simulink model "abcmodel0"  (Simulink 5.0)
settings: Solver=ode45  StartTime=0.0  StopTime=2  RelTol=1e-3
InitFcn:
  | imparamsim0
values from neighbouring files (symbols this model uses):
  Bm = 0.10    (= 0.1)    [IMabc2.m]    (also in imabcparam.m = 0.01; IMabcrun0.m = 0.01; IMabcrun1.m = 0.001; IMcur0.m = 1e-06)
  gam = 2*pi/3    (= 2.09439510239)    [IMabc2.m]    (also in IMabcf0.m; IMabcf1.m; imabcparam.m; IMabcrun0.m)
  J = 0.02    [imabcparam.m]    (also in IMabcrun0.m; IMabcrun1.m; imdefSIvec1.m = 0.03)
  Lm1 = 2/3*Lm    [IMabcf0.m]    (also in IMabcf1.m; imabcparam.m = 0.0564666666667; IMabcrun0.m = 0.0564666666667; IMabcrun1.m = 0.0564666666667)
  Lrr = [Lr   -Lm/2 -Lm/2    [IMabc2.m]    (also in IMabcf0.m = [Lr   -Lm1/2 -Lm1/2; IMabcf1.m = [Lr   -Lm1/2 -Lm1/2)
  Lss = [Ls   -Lm/2 -Lm/2    [IMabc2.m]    (also in IMabcf0.m = [Ls   -Lm1/2 -Lm1/2; IMabcf1.m = [Ls   -Lm1/2 -Lm1/2)
  nsync = 120*freq0/p    (= 1800)    [imabcparam.m]
  p = cos(beta-alpha)    [abcRwdg.m]    (also in alternator.m = 0:pi/20:2*pi; altwdgs.m = 0:pi/20:2*pi; brushlessdcB.m = 0:pi/100:2*pi; brushlessdcnew.m = 0:pi/100:2*pi)
  R = str2num(get(h,'string'))    [acttrcalc1.m]    (also in IMabc2.m = diag([Rs Rs Rs Rr Rr Rr]); IMabcf0.m = diag([Rs Rs Rs Rr Rr Rr]); IMabcf1.m = diag([Rs Rs Rs Rr Rr Rr]); IMcurf0.m = diag([Rs Rs Rr Rr]))
  Vs = abs(Vas)    [calc0.m]    (also in Ccurverun.m = 1; IMabc2.m = 1; IMabcrun0.m = Vll*sqrt(2/3); IMabcrun1.m = Vll*sqrt(2/3))
  wk = ws    (= 1)    [imdef0vec.m]    (also in imdef1vec.m; imdef2vec.m; imdefrotflux.m; imdefSIvec1.m)
  wo = 2*pi*freq0    [calc0.m]    (also in IMabc2.m = 376.991118431; imabcparam.m = 376.991118431; IMabcrun0.m = 376.991118431; IMabcrun1.m = 376.991118431)
undefined symbols (not defined in the file or in its folder): TL1, TL2
libraries: simulink x17

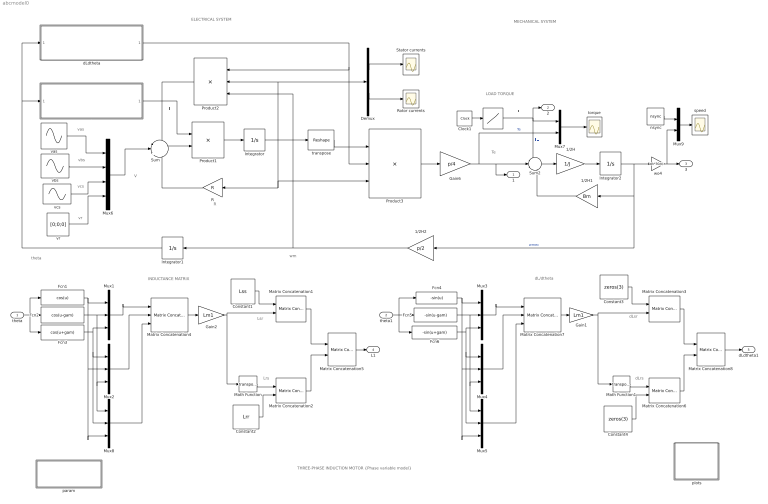
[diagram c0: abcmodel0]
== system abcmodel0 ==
  note: I
  note: I'
  note: MECHANICAL SYSTEM
  note: ELECTRICAL SYSTEM
  note: V
  note: theta
  note: THREE-PHASE INDUCTION MOTOR {Phase variable model}
  note: L
  note: Te
  note: LOAD TORQUE
  note: TL
  note: wm
  note: Lrs
  note: Lsr
  note: INDUCTANCE MATRIX
  note: dLrs
  note: dLsr
  note: dL/dtheta
  note: R
  note: vas
  note: vbs
  note: vcs
  note: vr
  theta : Inport
  theta1 : Inport  Port=2
  " " : Lookup  InputValues=[0 0.6 0.6 1.4 1.4 2]  OutputValues="[TL1 TL1  TL2 TL2 TL1 TL1]"
  1/2H : Gain  Gain=1/J
  1/2H1 : Gain  Orientation=left  Gain=Bm
  1/2H2 : Gain  Orientation=left  Gain=p/2
  Clock1 : Clock
  Constant1 : Constant  Value=Lss  VectorParams1D=off
  Constant2 : Constant  Value=Lrr  VectorParams1D=off
  Constant3 : Constant  Value=zeros(3)  VectorParams1D=off
  Constant4 : Constant  Value=zeros(3)  VectorParams1D=off
  Demux : Demux  Outputs=2
  Fcn1 : Fcn  Expr=cos(u)
  Fcn2 : Fcn  Expr=cos(u-gam)
  Fcn3 : Fcn  Expr=cos(u+gam)
  Fcn4 : Fcn  Expr=-sin(u)
  Fcn5 : Fcn  Expr=-sin(u-gam)
  Fcn6 : Fcn  Expr=-sin(u+gam)
  Gain1 : Gain  Gain=Lm1
  Gain2 : Gain  Gain=Lm1
  Gain6 : Gain  Gain=p/4  ShowAdditionalParam=on
  Integrator : Integrator  InitialCondition=[0 ;0 ;0; 0 ;0 ;0]
  Integrator1 : Integrator  Orientation=left
  Integrator2 : Integrator  InitialCondition=wo*2/p
  L : Subsystem
  Math Function : Math  Operator=transpose
  Math Function1 : Math  Operator=transpose
  Matrix Concatenation{1..3,6} (4 alike) : simulink/Math Operations/Matrix Concatenation  numInports=2  catMethod=Horizontal
  Matrix Concatenation4 : simulink/Math Operations/Matrix Concatenation  numInports=3  catMethod=Horizontal
  Matrix Concatenation5 : simulink/Math Operations/Matrix Concatenation  numInports=2  catMethod=Vertical
  Matrix Concatenation7 : simulink/Math Operations/Matrix Concatenation  numInports=3  catMethod=Horizontal
  Matrix Concatenation8 : simulink/Math Operations/Matrix Concatenation  numInports=2  catMethod=Vertical
  Mux{1..5,8} (6 alike) : Mux  Inputs=3
  Mux6 : Mux
  Mux7 : Mux  Inputs=2
  Mux9 : Mux  Inputs=2
  Product1 : Product  Inputs=/*  Multiplication=Matrix(*)
  Product2 : Product  Orientation=left  Inputs=***  Multiplication=Matrix(*)
  Product3 : Product  Inputs=3  Multiplication=Matrix(*)  ShowAdditionalParam=on
  R : Gain  Orientation=left  Gain=R  Multiplication=Matrix(K*u)
  Rotor currents : Scope
  Stator currents : Scope
  Sum : Sum  Inputs=-|+|-
  Sum2 : Sum  Inputs=-+-
  dLdtheta : Subsystem
  nsync : Constant  Value=nsync
  param : Subsystem
  plots : Subsystem
  speed : Scope
  torque : Scope
  transpose : simulink/Math Operations/Reshape  OutputDimensionality=Row vector  OutputDimensions=[1,6]
  vas : Sin  Amplitude=Vs  Frequency=wo  Phase=pi/2  SampleTime=0
  vbs : Sin  Amplitude=Vs  Frequency=wo  Phase=pi/2-gam  SampleTime=0
  vcs : Sin  Amplitude=Vs  Frequency=wo  Phase=pi/2+gam  SampleTime=0
  vr : Constant  Value=[0;0;0]  VectorParams1D=off
  wo4 : Gain  Gain=wk*30/pi
  1 : Outport
  2 : Outport  Port=2
  3 : Outport  Port=3
  L1 : Outport  Port=4
  dLdtheta1 : Outport  Port=5
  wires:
  Product1/1 -> Integrator/1
  Integrator/1 -> Product3/3, R/1, transpose/1, Product2/2, Demux/1
  Sum/1 -> Product1/2
  R/1 -> Sum/3
  transpose/1 -> Product3/1
  Demux/1 -> Stator currents/1
  Demux/2 -> Rotor currents/1
  Product2/1 -> Sum/1
  dLdtheta/1(dLdtheta) -> Product2/1, Product3/2
  Product3/1 -> Gain6/1
  Mux6/1 -> Sum/2
  L/1(L) -> Product1/1
  vbs/1 -> Mux6/2
  vas/1 -> Mux6/1
  vr/1 -> Mux6/4
  Sum2/1 -> 1/2H/1
  1/2H/1 -> Integrator2/1
  1/2H1/1 -> Sum2/3
  wo4/1 -> Mux9/2, 3/1
  Mux9/1 -> speed/1
  nsync/1 -> Mux9/1
  Mux7/1 -> torque/1
  " "/1 -> Mux7/1, Sum2/1, 2/1  "TL"
  Gain6/1 -> Sum2/2, 1/1, Mux7/2  "Te"
  Integrator2/1 -> wo4/1, 1/2H1/1, 1/2H2/1  "wmec"
  1/2H2/1 -> Integrator1/1, Product2/3
  Clock1/1 -> " "/1
  Integrator1/1 -> dLdtheta/1(theta1), L/1(theta)
  Fcn1/1 -> Mux1/1, Mux2/2, Mux8/3
  Fcn2/1 -> Mux8/1, Mux2/3, Mux1/2
  Fcn3/1 -> Mux8/2, Mux2/1, Mux1/3
  Constant2/1 -> Matrix Concatenation2/2
  Constant1/1 -> Matrix Concatenation1/1
  Matrix Concatenation2/1 -> Matrix Concatenation5/2
  Matrix Concatenation1/1 -> Matrix Concatenation5/1
  Mux2/1 -> Matrix Concatenation4/2
  Mux8/1 -> Matrix Concatenation4/3
  Matrix Concatenation4/1 -> Gain2/1
  Mux1/1 -> Matrix Concatenation4/1
  Gain2/1 -> Math Function/1, Matrix Concatenation1/2
  Math Function/1 -> Matrix Concatenation2/1
  theta/1 -> Fcn2/1, Fcn1/1, Fcn3/1
  Matrix Concatenation5/1 -> L1/1
  Matrix Concatenation8/1 -> dLdtheta1/1
  Fcn4/1 -> Mux3/1, Mux4/2, Mux5/3
  Fcn5/1 -> Mux5/1, Mux4/3, Mux3/2
  Fcn6/1 -> Mux5/2, Mux4/1, Mux3/3
  Constant4/1 -> Matrix Concatenation6/2
  Constant3/1 -> Matrix Concatenation3/1
  Matrix Concatenation6/1 -> Matrix Concatenation8/2
  Matrix Concatenation3/1 -> Matrix Concatenation8/1
  Mux4/1 -> Matrix Concatenation7/2
  Mux5/1 -> Matrix Concatenation7/3
  Matrix Concatenation7/1 -> Gain1/1
  Mux3/1 -> Matrix Concatenation7/1
  Gain1/1 -> Math Function1/1, Matrix Concatenation3/2
  Math Function1/1 -> Matrix Concatenation6/1
  theta1/1 -> Fcn6/1, Fcn5/1, Fcn4/1
  vcs/1 -> Mux6/3

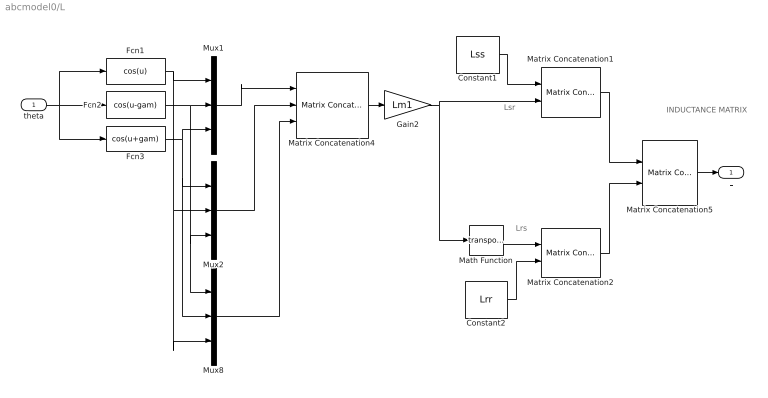
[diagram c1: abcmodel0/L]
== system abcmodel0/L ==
  note: Lrs
  note: Lsr
  note: INDUCTANCE MATRIX
  theta : Inport
  Constant1 : Constant  Value=Lss  VectorParams1D=off
  Constant2 : Constant  Value=Lrr  VectorParams1D=off
  Fcn1 : Fcn  Expr=cos(u)
  Fcn2 : Fcn  Expr=cos(u-gam)
  Fcn3 : Fcn  Expr=cos(u+gam)
  Gain2 : Gain  Gain=Lm1
  Math Function : Math  Operator=transpose
  Matrix Concatenation1 : simulink/Math Operations/Matrix Concatenation  numInports=2  catMethod=Horizontal
  Matrix Concatenation2 : simulink/Math Operations/Matrix Concatenation  numInports=2  catMethod=Horizontal
  Matrix Concatenation4 : simulink/Math Operations/Matrix Concatenation  numInports=3  catMethod=Horizontal
  Matrix Concatenation5 : simulink/Math Operations/Matrix Concatenation  numInports=2  catMethod=Vertical
  Mux1 : Mux  Inputs=3
  Mux2 : Mux  Inputs=3
  Mux8 : Mux  Inputs=3
  L : Outport
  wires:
  Fcn1/1 -> Mux1/1, Mux2/2, Mux8/3
  Fcn2/1 -> Mux8/1, Mux2/3, Mux1/2
  Fcn3/1 -> Mux8/2, Mux2/1, Mux1/3
  Constant2/1 -> Matrix Concatenation2/2
  Constant1/1 -> Matrix Concatenation1/1
  Matrix Concatenation2/1 -> Matrix Concatenation5/2
  Matrix Concatenation1/1 -> Matrix Concatenation5/1
  Mux2/1 -> Matrix Concatenation4/2
  Mux8/1 -> Matrix Concatenation4/3
  Matrix Concatenation4/1 -> Gain2/1
  Mux1/1 -> Matrix Concatenation4/1
  Gain2/1 -> Math Function/1, Matrix Concatenation1/2
  Math Function/1 -> Matrix Concatenation2/1
  theta/1 -> Fcn2/1, Fcn1/1, Fcn3/1
  Matrix Concatenation5/1 -> L/1

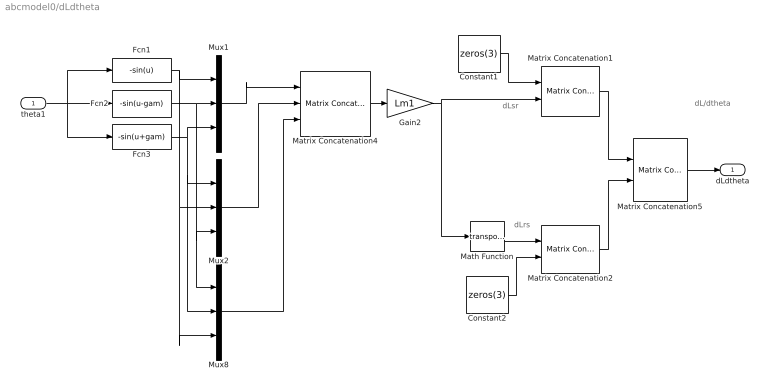
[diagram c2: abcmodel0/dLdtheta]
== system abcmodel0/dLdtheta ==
  note: dLrs
  note: dLsr
  note: dL/dtheta
  theta1 : Inport
  Constant1 : Constant  Value=zeros(3)  VectorParams1D=off
  Constant2 : Constant  Value=zeros(3)  VectorParams1D=off
  Fcn1 : Fcn  Expr=-sin(u)
  Fcn2 : Fcn  Expr=-sin(u-gam)
  Fcn3 : Fcn  Expr=-sin(u+gam)
  Gain2 : Gain  Gain=Lm1
  Math Function : Math  Operator=transpose
  Matrix Concatenation1 : simulink/Math Operations/Matrix Concatenation  numInports=2  catMethod=Horizontal
  Matrix Concatenation2 : simulink/Math Operations/Matrix Concatenation  numInports=2  catMethod=Horizontal
  Matrix Concatenation4 : simulink/Math Operations/Matrix Concatenation  numInports=3  catMethod=Horizontal
  Matrix Concatenation5 : simulink/Math Operations/Matrix Concatenation  numInports=2  catMethod=Vertical
  Mux1 : Mux  Inputs=3
  Mux2 : Mux  Inputs=3
  Mux8 : Mux  Inputs=3
  dLdtheta : Outport
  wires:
  Matrix Concatenation5/1 -> dLdtheta/1
  Fcn1/1 -> Mux1/1, Mux2/2, Mux8/3
  Fcn2/1 -> Mux8/1, Mux2/3, Mux1/2
  Fcn3/1 -> Mux8/2, Mux2/1, Mux1/3
  Constant2/1 -> Matrix Concatenation2/2
  Constant1/1 -> Matrix Concatenation1/1
  Matrix Concatenation2/1 -> Matrix Concatenation5/2
  Matrix Concatenation1/1 -> Matrix Concatenation5/1
  Mux2/1 -> Matrix Concatenation4/2
  Mux8/1 -> Matrix Concatenation4/3
  Matrix Concatenation4/1 -> Gain2/1
  Mux1/1 -> Matrix Concatenation4/1
  Gain2/1 -> Math Function/1, Matrix Concatenation1/2
  Math Function/1 -> Matrix Concatenation2/1
  theta1/1 -> Fcn3/1, Fcn2/1, Fcn1/1

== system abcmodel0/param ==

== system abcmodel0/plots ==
